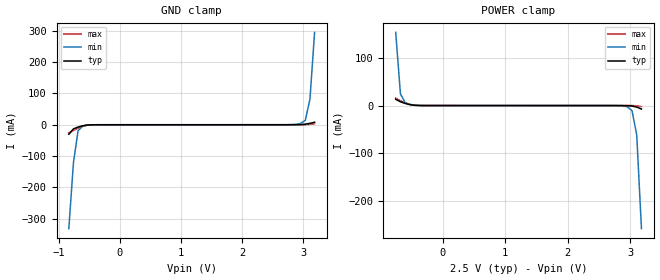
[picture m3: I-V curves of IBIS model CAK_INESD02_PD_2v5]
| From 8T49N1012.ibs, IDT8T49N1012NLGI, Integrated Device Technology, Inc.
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[Model] CAK_INESD02_PD_2v5
Model_type   Input
Polarity   Non-Inverting
Vinl = 0.7V
Vinh = 1.7V
|   typ   min   max
C_comp   2pF   1.5pF   2.5pF
|   typ   min   max
[Voltage range]   2.5V   2.375V   2.625V
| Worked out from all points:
|   GND clamp passes 1 mA (typ) near -0.53 V on its own axis
|   POWER clamp passes 1 mA (typ) near -0.48 V on its own axis
[GND_clamp]
|Voltage   I (typ)   I (min)   I (max)
|Note, modeling breaks down at 250mA and above.  This is well beyond the functional   |
|operating range of the device.  Should this scenario occur, catastrophic failure and   |
|possible damage to the device and/or board is of higher concern than the I-V curve   |
|behavior.  The IBIS checker will flag currents in excess of 10A with warnings.  Lines   |
|with currents in excess of 0.35 A have been commented out.  The points still remain|
|available to the user if the user desires to use them.   |
|-2.50000e+00   -6.16885e+00   -5.01107e+00   -7.48547e+00
|-2.42424e+00   -5.88381e+00   -4.79760e+00   -7.12142e+00
|-2.34848e+00   -5.59879e+00   -4.58417e+00   -6.75739e+00
|-2.27273e+00   -5.31381e+00   -4.37080e+00   -6.39336e+00
|-2.19697e+00   -5.02886e+00   -4.15748e+00   -6.02935e+00
|-2.12121e+00   -4.74395e+00   -3.94422e+00   -5.66536e+00
|-2.04545e+00   -4.45909e+00   -3.73102e+00   -5.30140e+00
|-1.96970e+00   -4.17427e+00   -3.51788e+00   -4.93748e+00
|-1.89394e+00   -3.88952e+00   -3.30482e+00   -4.57359e+00
|-1.81818e+00   -3.60483e+00   -3.09183e+00   -4.20976e+00
|-1.74242e+00   -3.32022e+00   -2.87892e+00   -3.84599e+00
|-1.66667e+00   -3.03569e+00   -2.66609e+00   -3.48227e+00
|-1.59091e+00   -2.75125e+00   -2.45335e+00   -3.11862e+00
|-1.51515e+00   -2.46691e+00   -2.24070e+00   -2.75504e+00
|-1.43939e+00   -2.18269e+00   -2.02814e+00   -2.39155e+00
|-1.36364e+00   -1.89859e+00   -1.81568e+00   -2.02815e+00
|-1.28788e+00   -1.61464e+00   -1.60332e+00   -1.66488e+00
|-1.21212e+00   -1.33083e+00   -1.39107e+00   -1.30175e+00
|-1.13636e+00   -1.04719e+00   -1.17894e+00   -9.38778e-01
|-1.06061e+00   -7.63732e-01   -9.66930e-01   -5.75993e-01
|-9.84848e-01   -4.80463e-01   -7.55072e-01   -2.13418e-01
|-9.09091e-01   -1.97405e-01   -5.43409e-01   -3.75925e-02
-833.3mV  -30.48mA   -332mA     -25.57mA
-757.6mV  -13.29mA   -120.7mA   -18.47mA
-681.8mV  -7.319mA   -19.01mA   -10.99mA
-606.1mV  -3.233mA   -4.077mA   -4.992mA
-530.3mV  -937.5uA   -1.009mA   -1.406mA
-378.8mV  -23.92uA   -40.87uA   -24.06uA
2.727V    54.58uA    114.9uA    62.76uA
2.955V    587.4uA    4.126mA    77.85uA
3.03V     1.971mA    14.15mA    222.3uA
3.106V    4.426mA    81.59mA    1.161mA
3.182V    7.979mA    295.1mA    3.423mA
| 3.25758e+00   1.31529e-02   5.12413e-01   7.00683e-03
| 3.33333e+00   3.25558e-02   7.29708e-01   1.18491e-02
| 3.40909e+00   2.27248e-01   9.47117e-01   1.71853e-02
| 3.48485e+00   5.17390e-01   1.16466e+00   2.19649e-02
| 3.56061e+00   8.07707e-01   1.38235e+00   5.22942e-02
| 3.63636e+00   1.09821e+00   1.60018e+00   3.65974e-01
| 3.71212e+00   1.38891e+00   1.81815e+00   7.37310e-01
| 3.78788e+00   1.67980e+00   2.03626e+00   1.10889e+00
| 3.86364e+00   1.97088e+00   2.25452e+00   1.48070e+00
| 3.93939e+00   2.26214e+00   2.47291e+00   1.85275e+00
| 4.01515e+00   2.55358e+00   2.69145e+00   2.22502e+00
| 4.09091e+00   2.84520e+00   2.91013e+00   2.59752e+00
| 4.16667e+00   3.13699e+00   3.12895e+00   2.97022e+00
| 4.24242e+00   3.42896e+00   3.34791e+00   3.34313e+00
| 4.31818e+00   3.72108e+00   3.56701e+00   3.71624e+00
| 4.39394e+00   4.01338e+00   3.78625e+00   4.08955e+00
| 4.46970e+00   4.30584e+00   4.00564e+00   4.46304e+00
| 4.54545e+00   4.59845e+00   4.22517e+00   4.83671e+00
| 4.62121e+00   4.89123e+00   4.44484e+00   5.21056e+00
| 4.69697e+00   5.18417e+00   4.66467e+00   5.58459e+00
| 4.77273e+00   5.47727e+00   4.88464e+00   5.95879e+00
| 4.84848e+00   5.77052e+00   5.10477e+00   6.33315e+00
| 4.92424e+00   6.06394e+00   5.32505e+00   6.70768e+00
| 5.00000e+00   6.35751e+00   5.54550e+00   7.08237e+00
[Power_clamp]
|Voltage   I (typ)   I (min)   I (max)
|Note, modeling breaks down at 250mA and above.  This is well beyond the functional   |
|operating range of the device.  Should this scenario occur, catastrophic failure and   |
|possible damage to the device and/or board is of higher concern than the I-V curve   |
|behavior.  The IBIS checker will flag currents in excess of 10A with warnings.  Lines   |
|with currents in excess of 0.35 A have been commented out.  The points still remain|
|available to the user if the user desires to use them.   |
|-2.50000e+00   6.35751e+00   5.18185e+00   7.70096e+00
|-2.42424e+00   6.06394e+00   4.96167e+00   7.32600e+00
|-2.34848e+00   5.77052e+00   4.74164e+00   6.95121e+00
|-2.27273e+00   5.47727e+00   4.52176e+00   6.57657e+00
|-2.19697e+00   5.18417e+00   4.30204e+00   6.20210e+00
|-2.12121e+00   4.89123e+00   4.08246e+00   5.82780e+00
|-2.04545e+00   4.59845e+00   3.86302e+00   5.45366e+00
|-1.96970e+00   4.30584e+00   3.64373e+00   5.07970e+00
|-1.89394e+00   4.01338e+00   3.42458e+00   4.70591e+00
|-1.81818e+00   3.72108e+00   3.20557e+00   4.33230e+00
|-1.74242e+00   3.42896e+00   2.98670e+00   3.95887e+00
|-1.66667e+00   3.13699e+00   2.76797e+00   3.58563e+00
|-1.59091e+00   2.84520e+00   2.54939e+00   3.21259e+00
|-1.51515e+00   2.55358e+00   2.33094e+00   2.83975e+00
|-1.43939e+00   2.26214e+00   2.11264e+00   2.46712e+00
|-1.36364e+00   1.97088e+00   1.89447e+00   2.09470e+00
|-1.28788e+00   1.67980e+00   1.67645e+00   1.72251e+00
|-1.21212e+00   1.38891e+00   1.45857e+00   1.35054e+00
|-1.13636e+00   1.09821e+00   1.24084e+00   9.78807e-01
|-1.06061e+00   8.07707e-01   1.02324e+00   6.07315e-01
|-9.84848e-01   5.17390e-01   8.05786e-01   2.36063e-01
|-9.09091e-01   2.27248e-01   5.88457e-01   3.12732e-02
|-8.33333e-01   3.25558e-02   3.71180e-01   2.01178e-02
-757.6mV  13.15mA    153.4mA    15.4mA
-681.8mV  7.979mA    24.72mA    10.02mA
-606.1mV  4.426mA    6.032mA    5.604mA
-530.3mV  1.971mA    2.157mA    2.479mA
-303mV    61.45uA    63.63uA    70.85uA
2.727V    -4.595uA   -23.61uA   -2.354uA
2.955V    -163.8uA   -2.507mA   -9.601uA
3.03V     -937.5uA   -10.7mA    -49.93uA
3.106V    -3.233mA   -61.64mA   -435.2uA
3.182V    -7.319mA   -258.1mA   -2.353mA
